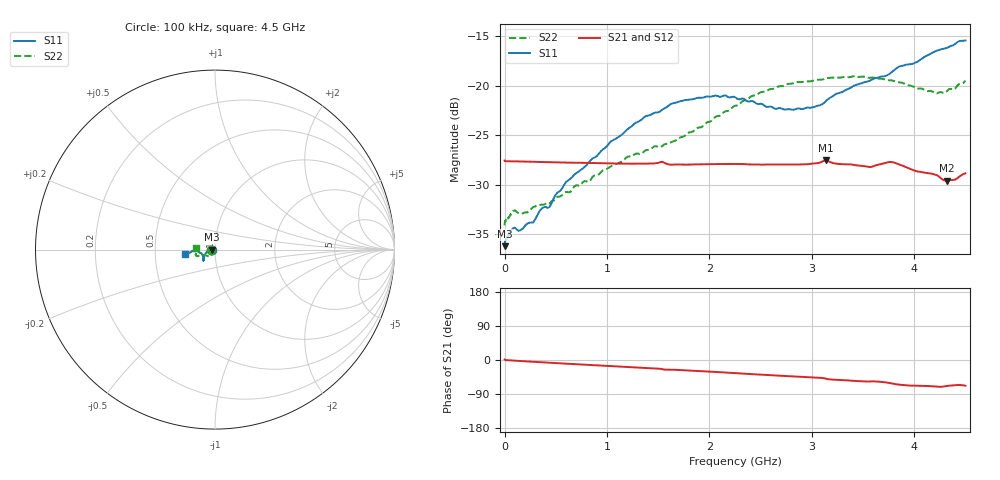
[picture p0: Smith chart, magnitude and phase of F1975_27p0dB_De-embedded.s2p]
! Integrated Device Technology
! Corporate Headquarters
! 6024 Silver Creek Valley Road
! San Jose, CA 95138  USA
! Phone:  1-408-284-8200
! Toll Free:  1-800-223-1366
! Webpage:  http://www.idt.com/
! Timing and RF Division
! 515 Groton Road, Suite 102
! Westford, MA 01886-6024
! Device:  F1975
! Description: 6-bit, 75 ohm, 0.5 dB Digital Step Attenuator
! Frequency:  5.0 MHz -  3.00 GHz
! Package:  4x4 mm QFN Plastic Package: 20 pin
! Ports:  2 RF, 11 DC
!  Pin  1  = D5 (16 dB)
!  Pin  2  = RF1  =  Port 1
!  Pin  3  = Serial Data In (DATA)
!  Pin  4  = Serial Clock (CLK)
!  Pin  5  = Serial Latch Enable (LE)
!  Pin  6  = VDD
!  Pin  7  = NC
!  Pin  8  = NC
!  Pin  9  = NC
!  Pin 10  = GND
!  Pin 11  = GND
!  Pin 12  = NC
!  Pin 13  = VMODE
!  Pin 14  = RF2  =  Port 2
!  Pin 15  = D4 (8 dB)
!  Pin 16  = D3 (4 dB)
!  Pin 17  = D2 (2 dB)
!  Pin 18  = NC
!  Pin 19  = D1 (1 dB)
!  Pin 20  = D0 (0.5 dB)
! State:  54
! Atten State:  27.0 dB
! Voltage:  +3.30 Volts
! Current:  0.590 mA
! Data:  The device was measured on a F1975 evaluation board which has
!  individual transmission lines to the RF pins.  Data was collected
!  using a calibrated network analyzer.  The evaluation board was
!  de-embedded using Automatic Fixture Removal (AFR).
!  The reference plane is the edge of the package pin.
! Misc:
!  Action Tracker AT0415
! Date Measured:  2018-02-08
! Date:  2018-03-26  MJV
! Note:
!  Integrated Device Technology supplies this data as a sample of measured
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# GHz S dB R 75
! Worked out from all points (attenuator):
!   291 points, 100 kHz to 4.5 GHz, reference 75 ohm
!   highest |S21| = -27.54 dB at 3.14 GHz (marker M1); lowest = -29.6 dB at 4.32 GHz (marker M2)
!   lowest |S11| = -36.2 dB at 100 kHz (marker M3), VSWR 1.03, Z = 72.7 - j0.0028 ohm
!   |S11| at or under -10 dB: start of sweep to end of sweep
!   |S22| runs from -34.1 to -19.0 dB; largest |S21 - S12| = 0.00014
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0.0001  -36.21 -179.9  -27.55 1.3  -27.56 1.2  -34.10 -179.2
0.006  -35.64 -178.2  -27.62 0.3  -27.62 0.3  -33.68 -177.9
0.08  -34.42 -176.4  -27.63 -1.4  -27.63 -1.4  -32.67 -169.1
0.16  -34.56 -177.6  -27.65 -2.8  -27.65 -2.8  -32.95 -159.4
0.28  -33.81 179.5  -27.68 -4.7  -27.67 -4.7  -32.25 -151.0
0.36  -32.44 179.5  -27.70 -6.0  -27.70 -6.0  -32.00 -143.5
0.44  -32.24 179.8  -27.72 -7.2  -27.72 -7.2  -31.90 -137.7
0.6  -29.72 -176.4  -27.76 -9.7  -27.76 -9.7  -30.72 -131.8
0.76  -28.38 -169.6  -27.79 -12.1  -27.79 -12.1  -29.78 -127.9
1.28  -23.74 -153.0  -27.87 -19.7  -27.87 -19.7  -26.86 -123.9
1.52  -22.58 -145.6  -27.71 -23.2  -27.71 -23.2  -26.21 -130.6
1.64  -21.78 -142.8  -27.97 -25.6  -27.97 -25.6  -25.64 -134.6
1.88  -21.22 -138.7  -27.94 -28.7  -27.94 -28.7  -24.27 -146.6
2.26  -21.21 -137.1  -27.90 -34.7  -27.89 -34.7  -22.00 -157.6
2.64  -22.32 -147.3  -27.95 -40.7  -27.95 -40.7  -20.25 -159.1
3.02  -22.15 -164.1  -27.84 -46.1  -27.84 -46.1  -19.46 -159.9
3.14  -21.52 -166.9  -27.54 -49.5  -27.53 -49.5  -19.23 -160.4
3.56  -19.51 -177.3  -28.20 -56.7  -28.20 -56.6  -19.20 -165.9
3.76  -18.79 -175.7  -27.70 -60.8  -27.70 -60.7  -19.45 -169.6
4.2  -16.54 -172.5  -28.97 -69.9  -28.96 -69.9  -20.76 178.9
4.32  -16.17 -171.9  -29.60 -68.6  -29.60 -68.6  -20.54 176.6
4.5  -15.42 -171.6  -28.85 -67.9  -28.84 -67.9  -19.48 173.9
